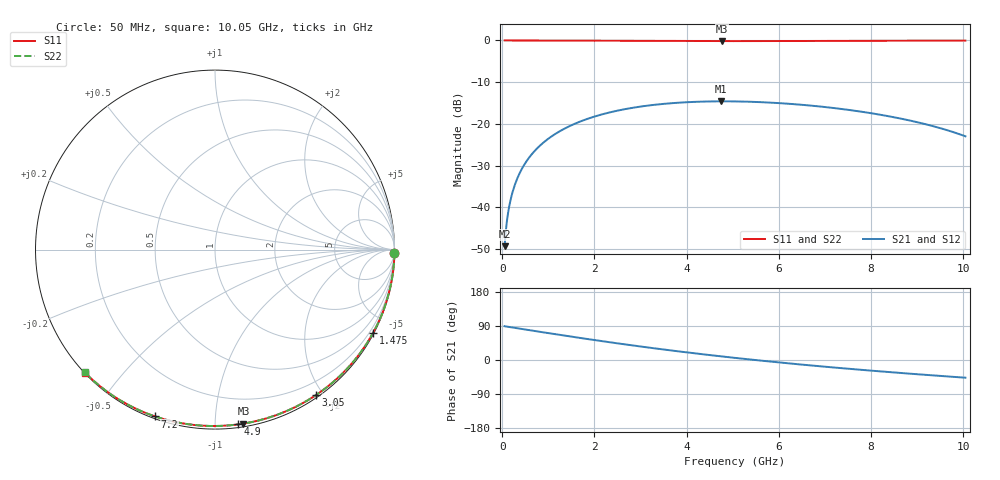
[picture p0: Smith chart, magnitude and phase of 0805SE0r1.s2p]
! AVX Thin Film Operation		Date: August 2001
! Description: Accu-P® Series, Thin Film, SMD, RF Capacitor
! Part Number: 08051J0R1ABT
! 50 MHz  -  10.05 GHz
! Serial Measurements
# mhz S db R 50
!	S11		S21		S12		S22
!	dB	Phase	dB	Phase	dB	Phase	dB	Phase
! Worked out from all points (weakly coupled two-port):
!   401 points, 50 MHz to 10.05 GHz, reference 50 ohm
!   highest |S21| = -14.59 dB at 4.75 GHz (marker M1); lowest = -49.3 dB at 50 MHz (marker M2)
!   lowest |S11| = -0.2 dB at 4.775 GHz (marker M3), VSWR 112.08, Z = 1.06 - j58.8 ohm
!   |S11| at or under -10 dB: nowhere
!   |S22| runs from -0.2 to 0.0 dB; largest |S21 - S12| = 0
!   S11 on the Smith chart (normalised r, x): 50 MHz: open; 1.475 GHz: 0.04, -4.03; 3.05 GHz: 0.03, -1.91; 4.9 GHz: 0.02, -1.14; 7.2 GHz: 0.01, -0.70; 10.05 GHz: 0.00, -0.40
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50  -0.00 -1.0  -49.32 89.2  -49.32 89.2  -0.00 -1.0
150  -0.00 -2.9  -39.78 87.1  -39.78 87.1  -0.00 -2.9
200  -0.00 -3.8  -37.29 86.2  -37.29 86.2  -0.00 -3.8
300  -0.00 -5.8  -33.77 84.2  -33.77 84.2  -0.00 -5.8
450  -0.00 -8.6  -30.28 81.4  -30.28 81.4  -0.00 -8.6
650  -0.01 -12.4  -27.14 77.6  -27.14 77.6  -0.01 -12.5
875  -0.01 -16.7  -24.65 73.3  -24.65 73.3  -0.01 -16.7
1150  -0.03 -21.9  -22.41 68.1  -22.41 68.1  -0.03 -21.9
1475  -0.04 -27.9  -20.46 62.1  -20.46 62.1  -0.04 -27.9
1725  -0.05 -32.4  -19.29 57.5  -19.29 57.5  -0.05 -32.5
2325  -0.08 -43.0  -17.26 46.9  -17.26 46.9  -0.08 -43.1
3050  -0.12 -55.2  -15.77 34.8  -15.77 34.8  -0.12 -55.2
3400  -0.13 -60.7  -15.31 29.3  -15.31 29.3  -0.13 -60.8
4750  -0.15 -80.4  -14.59 9.6  -14.59 9.6  -0.15 -80.4
4775  -0.15 -80.7  -14.59 9.2  -14.59 9.2  -0.15 -80.8
4900  -0.15 -82.4  -14.60 7.6  -14.60 7.6  -0.15 -82.4
5050  -0.15 -84.4  -14.61 5.6  -14.61 5.6  -0.15 -84.4
6725  -0.12 -104.6  -15.65 -14.7  -15.65 -14.7  -0.12 -104.7
7200  -0.11 -109.8  -16.21 -19.8  -16.21 -19.8  -0.11 -109.8
8400  -0.07 -121.9  -18.20 -31.9  -18.20 -31.9  -0.07 -121.9
9250  -0.04 -129.7  -20.26 -39.8  -20.26 -39.8  -0.04 -129.8
10050  -0.03 -136.6  -22.98 -46.7  -22.98 -46.7  -0.03 -136.7
